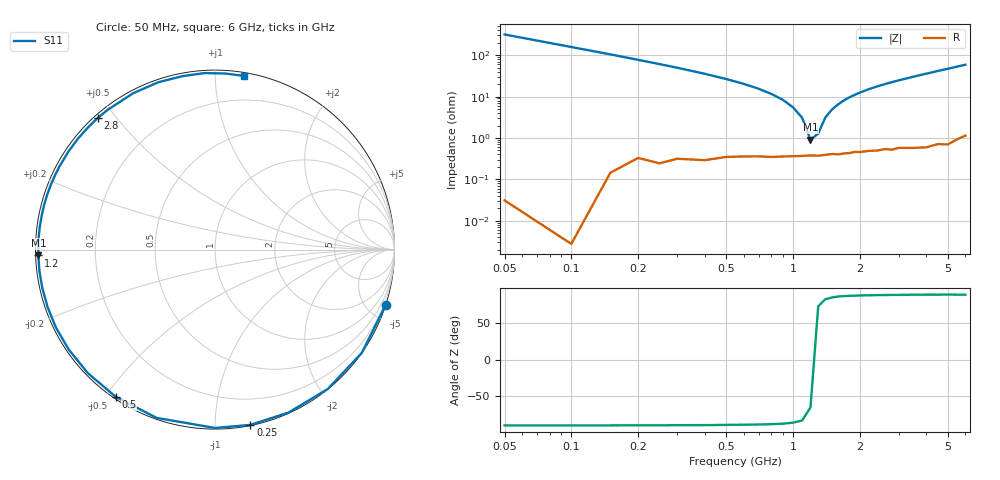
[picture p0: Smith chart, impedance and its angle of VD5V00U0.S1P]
! Infineon Technologies  Discrete & RF Semiconductors
! BBY 55-03
! Si Tuning Diode in SOD323
! VR = 5 V
! S-Parameters:  June  1999
# GHz  S  MA  R  50
!  f  S11
! GHz  MAG  ANG
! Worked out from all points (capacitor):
!   34 points, 50 MHz to 6 GHz, reference 50 ohm
!   read as one part to ground: C = 10 pF near 50 MHz
!   lowest |Z| = 912 mohm at 1.2 GHz (marker M1)
!   series resonance near 1.24 GHz, so ESL is about 1.6 nH
!   S11 on the Smith chart (normalised r, x): 50 MHz: 0.00, -6.35; 250 MHz: 0.00, -1.22; 500 MHz: 0.01, -0.53; 1.2 GHz: 0.01, -0.02; 2.8 GHz: 0.01, +0.45; 6 GHz: 0.02, +1.18
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0.05  1 -17.9
0.1  1 -35.1
0.15  0.9989 -51.0
0.2  0.9961 -65.7
0.25  0.9961 -78.6
0.3  0.9937 -90.0
0.4  0.9923 -109.1
0.5  0.9892 -124.0
0.6  0.9878 -135.8
0.7  0.987 -145.6
0.8  0.9869 -153.9
0.9  0.9862 -161.0
1  0.9857 -167.4
1.2  0.9849 -178.1
1.4  0.9846 172.9
1.6  0.9844 165.2
1.8  0.9835 158.2
2  0.9829 152.1
2.2  0.9823 146.3
2.4  0.9825 141.1
2.8  0.9827 131.7
3  0.9816 127.4
3.5  0.9833 117.6
4  0.9844 108.7
4.5  0.9833 100.6
5  0.9853 93.4
5.5  0.9827 86.6
6  0.9811 80.6
